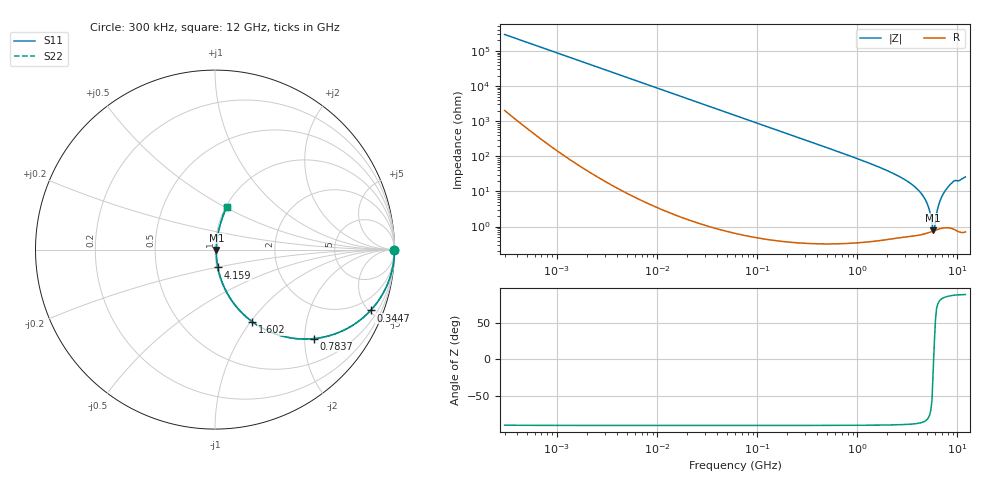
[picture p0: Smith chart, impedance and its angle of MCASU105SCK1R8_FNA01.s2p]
! MCASU105SCK1R8_FNA01  S-PARAMETER MODEL  ( Standard Model )
! Model Generated by TAIYO YUDEN Corporation (http://www.ty-top.com)
! Version 1.0
! TAIYO YUDEN Control No. 230609
! Copyright(c) 2023 TAIYO YUDEN CO.,LTD. All Rights Reserved.
! Product Description (link to TY-COMPAS)
! https://ds.yuden.co.jp/TYCOMPAS/or/detail?pn=MCASU105SCK1R8CFNA01&u=M
! Products Name : Multilayer Ceramic Capacitors
! Characteristics :
!  Capacitance : 1.8 [pF] , Rated Voltage : 50 [V] , TCC : CK / C0K
!  Case Size : 1.0 x 0.5 / 0.039 x 0.02 [mm/inch] , Thickness : 0.5 / 0.02 [mm/inch]
!  (Conditions: Temperature = 25 [degC] , DC Bias Voltage = 0 [V])
! External Node Assignments :
!  1  o---| |---o  2
! GND o---------o GND
! Frequency Range : 0.3MHz  -  12000MHz  [ 401 STEP ]
# MHZ S RI R 50
! Freq[MHz].  S11 Real  S11 Imag  S21 Real  S21 Imag  S12 Real  S12 Imag  S22 Real  S22 Imag
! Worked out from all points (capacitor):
!   401 points, 300 kHz to 12 GHz, reference 50 ohm
!   read as one part in series: C = 1.8 pF near 316.3 kHz
!   lowest |Z| = 779 mohm at 5.715 GHz (marker M1)
!   series resonance near 5.781 GHz, so ESL is about 420 pH
!   S11 on the Smith chart (normalised r, x): 300 kHz: open; 344.7 MHz: 1.01, -5.11; 783.7 MHz: 1.01, -2.21; 1.602 GHz: 1.01, -1.02; 4.159 GHz: 1.01, -0.20; 12 GHz: 1.01, +0.52
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0.3  1 -0.000339  2.44e-06 0.000339  2.44e-06 0.000339  1 -0.000339
1.769972  1 -0.002  5.95e-06 0.002  5.95e-06 0.002  1 -0.002
10.44266  0.9999 -0.0118  0.000144 0.0118  0.000144 0.0118  0.9999 -0.0118
60  0.9954 -0.0676  0.00461 0.0676  0.00461 0.0676  0.9954 -0.0676
177.7716  0.9609 -0.1934  0.0391 0.1934  0.0391 0.1934  0.9609 -0.1934
344.7396  0.8669 -0.339  0.1331 0.339  0.1331 0.339  0.8669 -0.339
353.9943  0.8606 -0.3457  0.1394 0.3457  0.1394 0.3457  0.8606 -0.3457
783.7017  0.5507 -0.4959  0.4493 0.4959  0.4493 0.4959  0.5507 -0.4959
1602.47  0.2076 -0.4018  0.7924 0.4018  0.7924 0.4018  0.2076 -0.4018
2088.533  0.122 -0.3214  0.878 0.3214  0.878 0.3214  0.122 -0.3214
3107.553  0.0436 -0.192  0.9564 0.192  0.9564 0.192  0.0436 -0.192
4158.869  0.0158 -0.0996  0.9842 0.0996  0.9842 0.0996  0.0158 -0.0996
4875.354  0.00895 -0.0507  0.9911 0.0507  0.9911 0.0507  0.00895 -0.0507
5140.631  0.00787 -0.0345  0.9921 0.0345  0.9921 0.0345  0.00787 -0.0345
5565.855  0.00732 -0.0104  0.9927 0.0104  0.9927 0.0104  0.00732 -0.0104
5715.274  0.00742 -0.00219  0.9926 0.00219  0.9926 0.00219  0.00742 -0.00219
6026.253  0.00795 0.0105  0.9921 -0.0105  0.9921 -0.0105  0.00795 0.0105
6354.153  0.00925 0.0313  0.9908 -0.0313  0.9908 -0.0313  0.00925 0.0313
6699.894  0.0114 0.0522  0.9886 -0.0522  0.9886 -0.0522  0.0114 0.0522
7648.807  0.0209 0.1073  0.9791 -0.1073  0.9791 -0.1073  0.0209 0.1073
9207.246  0.045 0.1873  0.955 -0.1873  0.955 -0.1873  0.045 0.1873
12000  0.0685 0.2393  0.9315 -0.2393  0.9315 -0.2393  0.0685 0.2393
